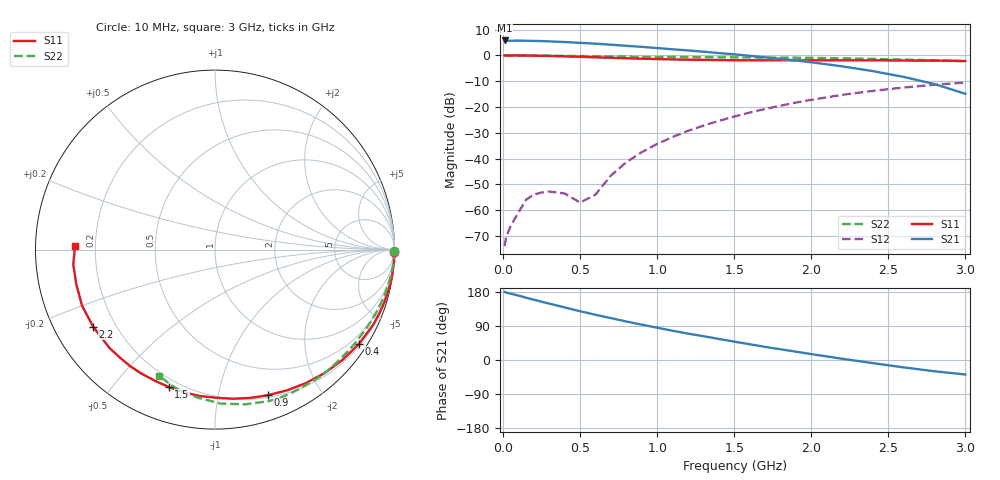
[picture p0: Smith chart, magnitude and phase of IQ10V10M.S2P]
! Infineon Technologies  Discrete & RF Semiconductors
! BF999
! Si MOSFET Triode in SOT23
! VDS = 10 V  ID = 10 mA
! Common Source S-Parameters:  October  2001
# GHz  S  MA  R  50
!  f  S11  S21  S12  S22
! GHz  MAG  ANG  MAG  ANG  MAG  ANG  MAG  ANG
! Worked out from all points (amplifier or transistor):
!   30 points, 10 MHz to 3 GHz, reference 50 ohm
!   highest |S21| = 5.8 dB at 10 MHz (marker M1)
!   |S21| within 3 dB of that: start of sweep to 1.01 GHz
!   unconditionally stable (mu >= 1): nowhere
!   at 200 MHz: K = 0.17, MSG = 29.8 dB, |S12| = -54.0 dB
!   at 1.1 GHz: K = -0.11, MSG = 17.0 dB, |S12| = -31.6 dB
!   at 3 GHz: K = 0.92, MSG = -2.2 dB, |S12| = -10.5 dB
!   S11 on the Smith chart (normalised r, x): 10 MHz: open; 400 MHz: 0.26, -3.33; 900 MHz: 0.22, -1.41; 1.5 GHz: 0.16, -0.71; 2.2 GHz: 0.12, -0.29; 3 GHz: 0.12, +0.01
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0.01  0.9999 -0.9  1.95 179.7  0.0002 110.2  0.9968 -0.4
0.02  0.9997 -1.7  1.917 178.2  0.0003 125.3  0.9964 -0.7
0.05  0.9994 -4.3  1.925 175.0  0.0005 85.6  0.997 -1.8
0.15  0.9931 -12.9  1.925 164.2  0.0016 78.6  0.9953 -5.5
0.2  0.9886 -17.0  1.909 159.2  0.002 79.4  0.9922 -7.3
0.25  0.9821 -21.2  1.897 153.8  0.0022 78.0  0.989 -9.1
0.3  0.9764 -25.3  1.871 148.7  0.0023 78.2  0.9863 -10.8
0.4  0.9585 -33.3  1.817 138.7  0.0021 80.9  0.9792 -14.3
0.5  0.9392 -41.0  1.752 128.7  0.0014 106.0  0.9719 -17.5
0.6  0.9192 -48.6  1.69 119.3  0.002 174.9  0.9649 -20.9
0.7  0.8999 -55.7  1.614 110.5  0.0047 -166.0  0.9578 -24.1
0.8  0.8815 -62.7  1.535 101.6  0.0085 -161.9  0.9502 -27.3
0.9  0.8634 -69.9  1.465 93.3  0.0133 -163.1  0.9436 -30.5
1.1  0.8367 -83.3  1.315 77.2  0.0262 -169.6  0.9329 -37.1
1.3  0.82 -96.0  1.181 62.8  0.0435 -176.5  0.924 -43.6
1.5  0.8076 -108.6  1.051 48.5  0.0652 175.5  0.9169 -50.9
1.6  0.8041 -114.3  0.983 41.6  0.0778 171.5  0.9109 -54.4
1.9  0.8016 -131.5  0.798 22.0  0.1217 159.1  0.902 -66.3
2.2  0.8033 -147.7  0.614 3.3  0.1717 145.7  0.8783 -79.0
2.4  0.8041 -157.1  0.496 -8.3  0.2055 136.7  0.858 -88.0
2.6  0.7966 -166.0  0.383 -19.5  0.2388 127.9  0.83 -96.9
3  0.7801 178.6  0.18 -38.3  0.298 111.8  0.7699 -114.0
